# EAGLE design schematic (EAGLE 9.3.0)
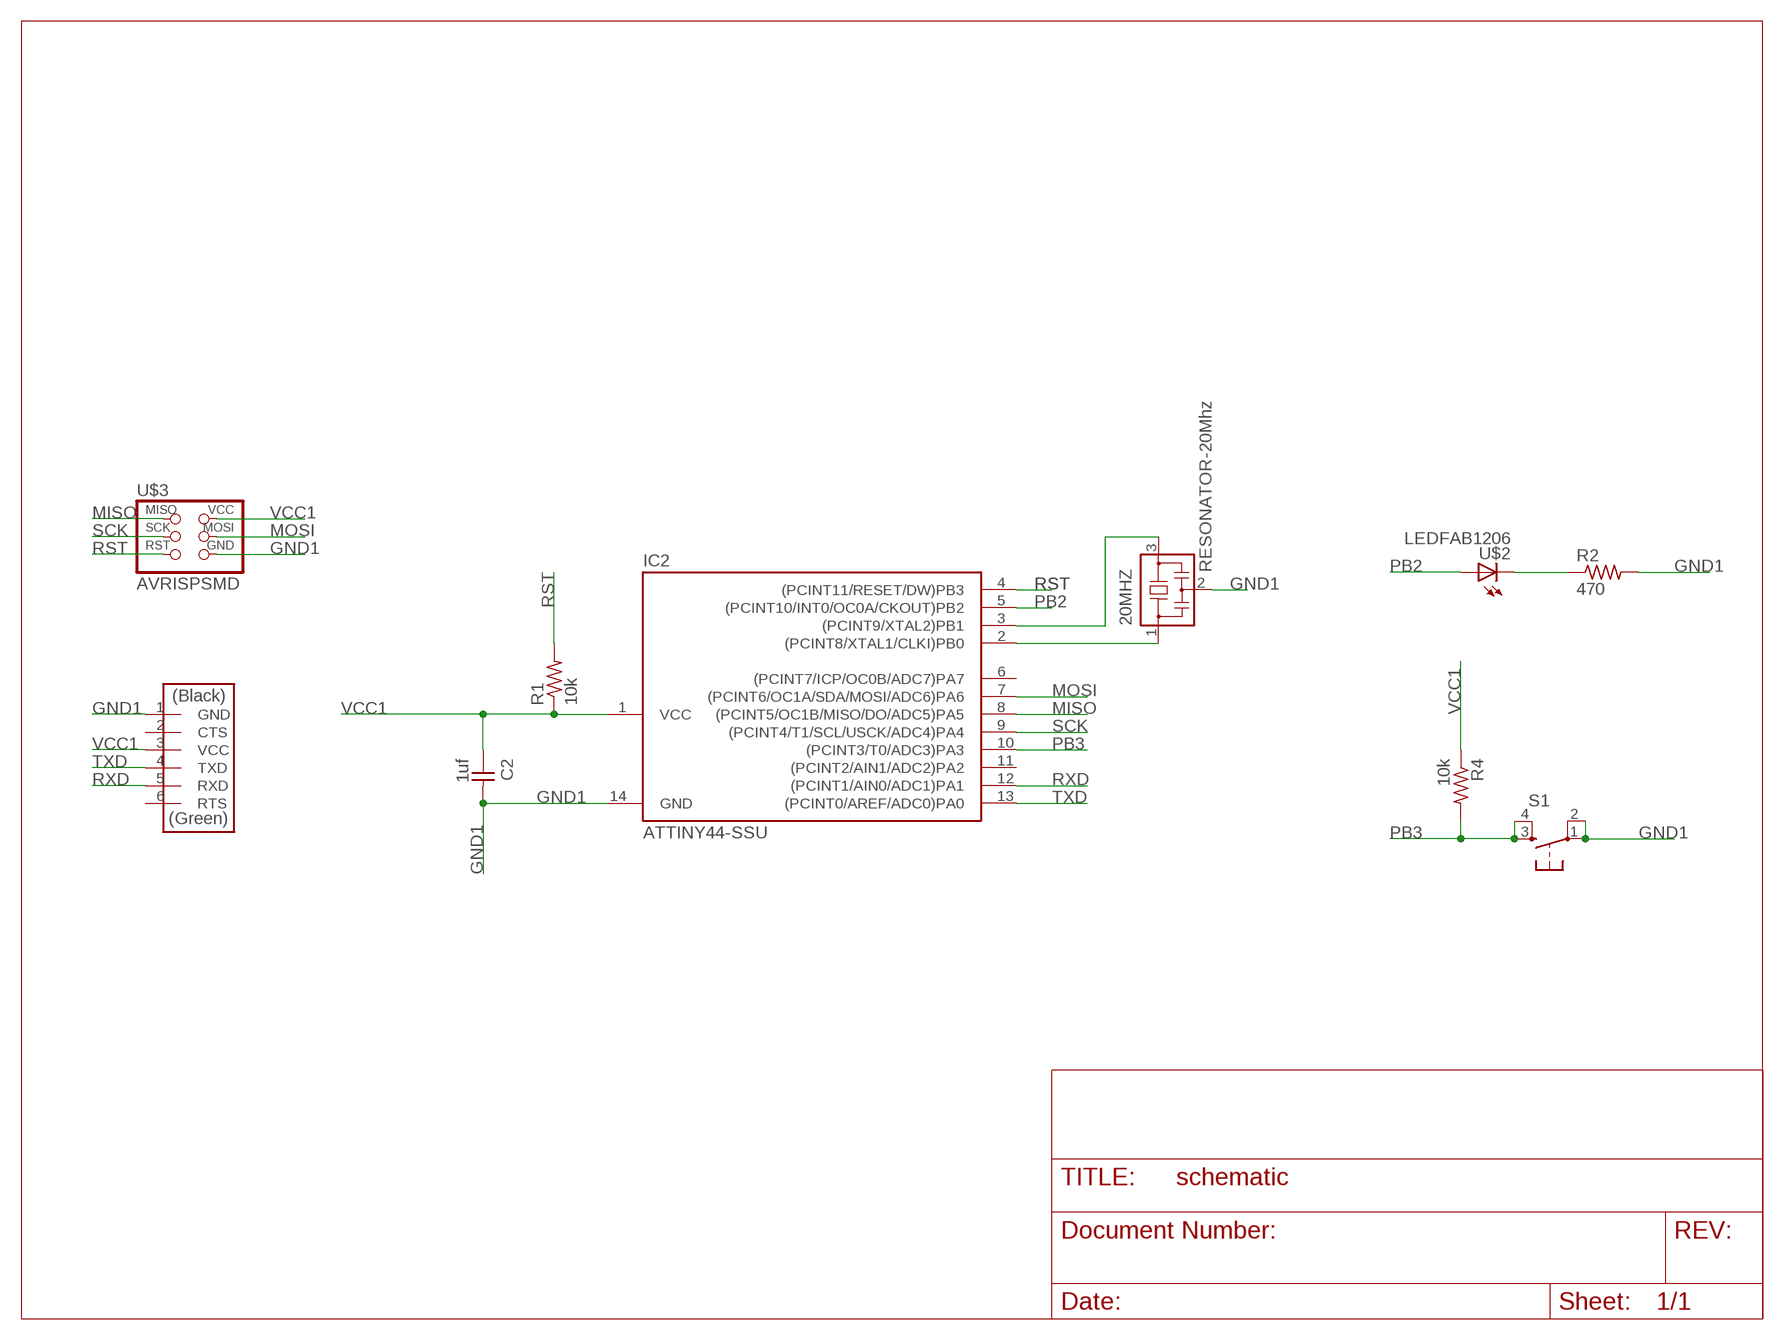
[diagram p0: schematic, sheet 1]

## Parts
20MHZ  RESONATOR-20Mhz  RESONATOR  [EFOBM]
C2  1uf  CAP-UNPOLARIZEDFAB  [C1206FAB]
IC2  ATTINY44-SSU  [SOIC14]
R1  10k  RES-US1206FAB  [R1206FAB]
R2  470  RES-US1206FAB  [R1206FAB]
R4  10k  RES-US1206FAB  [R1206FAB]
S1  switch 6mm  6MM_SWITCH6MM_SWITCH  [6MM_SWITCH]
U$1  FTDI-SMD-HEADER  [1X06SMD]
U$2  LEDFAB1206  [LED1206FAB]
U$3  AVRISPSMD  [2X03SMD]

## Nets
GND1: 20MHZ.2 C2.2 IC2.14(GND) R2.2 S1.1(P) S1.2(P1) U$1.1(GND) U$3.6(GND)
MISO: IC2.8((PCINT5/OC1B/MISO/DO/ADC5)PA5) U$3.1(MISO)
MOSI: IC2.7((PCINT6/OC1A/SDA/MOSI/ADC6)PA6) U$3.4(MOSI)
N$2: 20MHZ.1 IC2.2((PCINT8/XTAL1/CLKI)PB0)
N$3: 20MHZ.3 IC2.3((PCINT9/XTAL2)PB1)
N$4: R2.1 U$2.2(C)
PB2: IC2.5((PCINT10/INT0/OC0A/CKOUT)PB2) U$2.1(A)
PB3: IC2.10((PCINT3/T0/ADC3)PA3) R4.2 S1.3(S) S1.4(S1)
RST: IC2.4((PCINT11/RESET/DW)PB3) R1.2 U$3.5(RST)
RXD: IC2.12((PCINT1/AIN0/ADC1)PA1) U$1.5(RXD)
SCK: IC2.9((PCINT4/T1/SCL/USCK/ADC4)PA4) U$3.3(SCK)
TXD: IC2.13((PCINT0/AREF/ADC0)PA0) U$1.4(TXD)
VCC1: C2.1 IC2.1(VCC) R1.1 R4.1 U$1.3(VCC) U$3.2(VCC)
Unconnected: IC2.6((PCINT7/ICP/OC0B/ADC7)PA7) IC2.11((PCINT2/AIN1/ADC2)PA2) U$1.2(CTS) U$1.6(RTS)

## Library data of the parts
20MHZ = fab:RESONATOR
C2 = fab:CAP-UNPOLARIZED; C1: 10uf
IC2 = fab:ATTINY44
R1 R2 R4 = fab:RES-US: Resistor (US Symbol)
S1 = fab:6MM_SWITCH: OMRON SWITCH
U$1 = fab:FTDI-SMD-HEADER
U$2 = fab:LED: LED
U$3 = fab:AVRISP

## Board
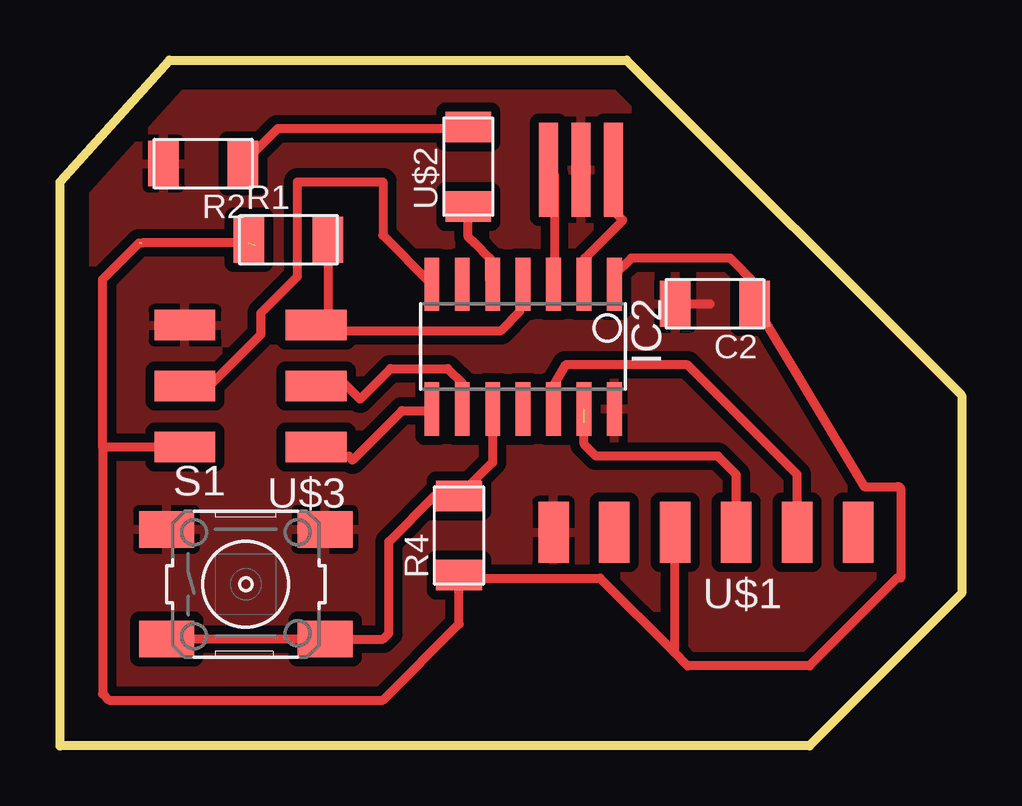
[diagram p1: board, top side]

Size 37.59 x 28.57 mm. Coordinates in mm from the lower left corner, seen from the top.
Outline: 31.24,0 0,0 0,23.5 4.57,28.57 23.62,28.57 37.59,14.61 37.59,6.35 31.24,0
Copper layers (1*16): Top 0.035mm / dielectric 1.5mm / Bottom 0.035mm
Design rules "CNC échoFab design rule 2X3": minimum track width 15mil, minimum drill 0.35mm, track to track 15mil, track to pad 15mil, pad to pad 6mil, via to via 6mil, smd to smd 6mil, copper to edge 40mil, drill to drill 6mil, minimum pad ring 10mil, minimum via ring 8mil, stop-mask expansion 4mil, vias tented up to drill 0mil, thermal gap 10mil

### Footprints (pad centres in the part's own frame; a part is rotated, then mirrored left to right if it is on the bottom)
EFOBM = smd 0.8 x 3.9: 1 -1.35,0; 2 0,0; 3 1.35,0
C1206FAB = smd 1.27 x 1.905: 1 -1.651,0; 2 1.651,0
SOIC14 = smd 0.61 x 2.21: 1 -3.81,-2.603; 2 -2.54,-2.603; 3 -1.27,-2.603; 4 0,-2.603; 5 1.27,-2.603; 6 2.54,-2.603; 7 3.81,-2.603; 8 3.81,2.603; 9 2.54,2.603; 10 1.27,2.603; 11 0,2.603; 12 -1.27,2.603; 13 -2.54,2.603; 14 -3.81,2.603
R1206FAB = smd 1.27 x 1.905: 1 -1.651,0; 2 1.651,0
6MM_SWITCH = smd 2.286 x 1.524: 1 -3.302,2.286; 2 3.302,2.286; 3 -3.302,-2.286; 4 3.302,-2.286
1X06SMD = smd 2.54 x 1.27: 1 0,6.35; 2 0,3.81; 3 0,1.27; 4 0,-1.27; 5 0,-3.81; 6 0,-6.35
LED1206FAB = smd 1.27 x 1.905: 1 -1.651,0; 2 1.651,0
2X03SMD = smd 2.54 x 1.27: 1 -2.54,2.54; 2 2.92,2.54; 3 -2.54,0; 4 2.92,0; 5 -2.54,-2.54; 6 2.92,-2.54

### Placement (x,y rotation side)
20MHZ  21.72,24 180 top
C2  27.3,18.41 180 top
IC2  19.3,16.64 180 top
R1  9.53,21.08 0 top
R2  5.97,24.26 180 top
R4  16.64,8.76 90 top
S1  7.75,6.73 0 top
U$1  26.92,8.89 90 top
U$2  17.02,24.13 90 top
U$3  8.13,14.99 180 top

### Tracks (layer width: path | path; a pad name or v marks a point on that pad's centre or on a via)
GND1
  Top 0.381: C2.2 27.11,18.41
  pour Top: 43.94,65.32 43.94,-3.18 4.57,-3.18 arc-90 -18.62,20.02
MISO
  Top 0.381: IC2.8 15.37,13.97 14.26,13.97 12.19,11.91 12.03,12.06 11.08,12.06 10.76,12.38 U$3.1
MOSI
  Top 0.381: IC2.7 13.46,21.27 13.46,23.5 9.91,23.5 9.91,19.56 8.38,18.03 8.38,17.14 6.22,14.99 U$3.4
N$2
  Top 0.381: IC2.2 21.88,19.37 21.88,20.32 23.46,21.91 23.15,22.23 23.15,23.97 20MHZ.1
N$3
  Top 0.381: IC2.3 20.61,19.37 20.61,23.81 20.45,23.97 20MHZ.3
N$4
  Top 0.381: U$2.2 16.95,25.72 9.08,25.72 R2.1
PB2
  Top 0.381: IC2.5 17.91,19.37 17.91,20.32 17.27,20.95 17.11,21.11 17.02,21.21 U$2.1
PB3
  Top 0.381: IC2.10 18.03,11.81 R4.2 15.62,10.41 13.72,8.51 13.72,4.7 13.46,4.45 S1.4 S1.3
RST
  Top 0.381: 10.76,17.62 U$3.5 | IC2.4 19.18,19.21 19.18,18.1 18.38,17.3 11.24,17.3 10.92,17.62 U$3.5 | R1.2 11.18,18.03 U$3.5
RXD
  Top 0.381: IC2.12 20.61,14.13 20.61,15.08 21.08,15.88 26.16,15.88 30.73,11.3 U$1.5
SCK
  Top 0.381: IC2.9 16.8,14.13 16.8,15.08 16.16,15.72 13.78,15.72 12.51,14.45 11.88,15.08 10.76,15.08 U$3.3
TXD  (1 unrouted)
  Top 0.381: 21.88,14.13 IC2.13 | 21.84,13.46 21.84,12.57 22.35,12.06 27.43,12.06 28.19,11.3 U$1.4
VCC1  (2 unrouted)
  Top 0.381: IC2.1 23.11,19.62 23.81,20.32 27.94,20.32 28.96,19.3 C2.1 33.53,10.79 34.93,10.79 arc-90 35.05,10.67 35.05,6.98 34.89,6.98 31.24,3.33 26.16,3.33 25.61,3.89 | 7.75,20.46 8.15,20.87 | 5.37,12.38 U$3.2 | 25.61,3.89 22.51,6.98 16.8,6.98 R4.1 16.64,5.08 13.46,1.9 2.03,1.9 1.78,2.16 1.78,12.45 | 5.37,12.22 U$3.2 | R1.1 7.87,20.95 3.43,20.95 | U$3.2 1.78,12.45 | 1.78,12.45 1.78,19.43 3.3,20.95 | U$1.3 25.61,8.84 25.61,3.89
